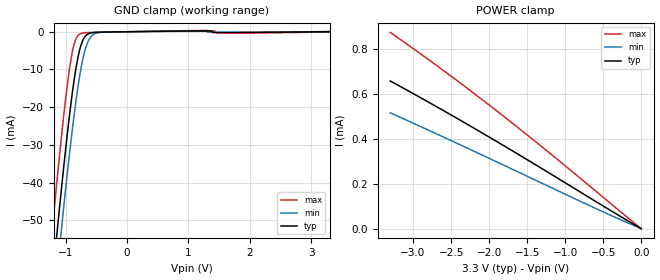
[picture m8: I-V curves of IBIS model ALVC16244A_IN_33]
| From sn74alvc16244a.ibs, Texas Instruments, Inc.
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[Model]   ALVC16244A_IN_33
Model_type  Input
Vinl=0.8
Vinh=2.0
| variable   typ   min   max
C_comp   0.96pF   0.60pF   1.24pF
[Temperature Range]   40   100   -40
| Ambient temperature   25   85   -40
[Voltage range]   3.3   3   3.6
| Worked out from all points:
|   GND clamp passes 1 mA (typ) near -0.67 V on its own axis
[GND Clamp]
| ALVC16244A_IN_33
|   Voltage   I(typ)   I(min)   I(max)
-3.3V     -452.1mA   -460.8mA   -441.7mA
-1.225V   -67.06mA   -77.83mA   -53.24mA
-1.14V    -52.82mA   -63.61mA   -38.94mA
-1.07V    -41.52mA   -52.25mA   -27.76mA
-985mV    -28.58mA   -39.06mA   -15.45mA
-905mV    -17.66mA   -27.51mA   -6.382mA
-845mV    -10.78mA   -19.68mA   -2.362mA
-765mV    -4.28mA    -10.91mA   -564.4uA
-705mV    -1.742mA   -6.047mA   -305uA
-635mV    -577uA     -2.546mA   -229.5uA
-470mV    -125.1uA   -255.7uA   -163.1uA
3.3V      1.116nA    43.97uA    -79.86uA
[POWER Clamp]
| ALVC16244A_IN_33
|   Voltage   I(typ)   I(min)   I(max)
-3.3V     655.9uA    514.6uA    871.8uA
-2.57V    518.5uA    402.2uA    694.9uA
-1.83V    373uA      285.5uA    504.7uA
-1.155V   235.8uA    177.9uA    322.3uA
-48.03fV  1.116nA    59.61nA    9.49pA
